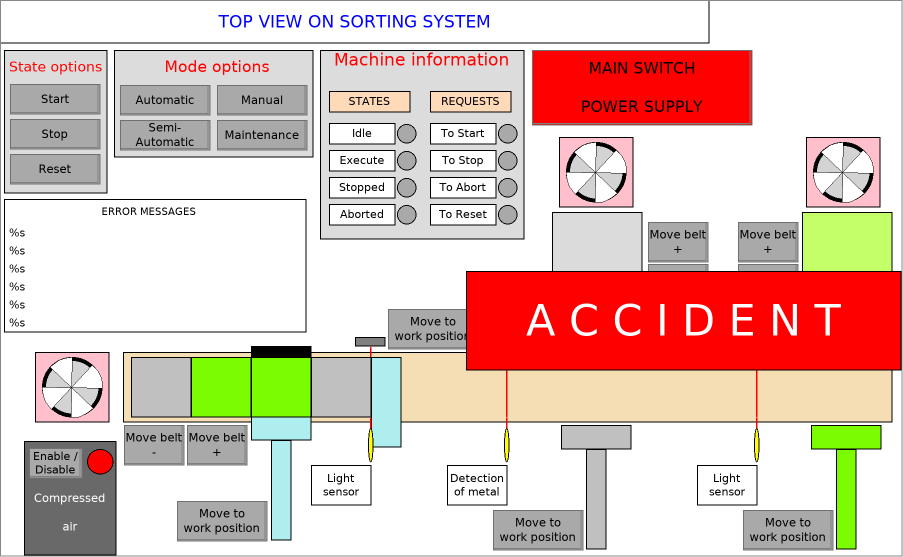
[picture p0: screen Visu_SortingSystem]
VISUALIZATION Visu_SortingSystem  // 903x557
    Rectangle (123,352 769x70)
    Rectangle (802,212 90x140)
    Rectangle (552,212 90x140)
    Rectangle (741,337 30x9)
    Rectangle (492,337 30x9)
    Ellipse (504,428 5x34)
    Ellipse (754,428 5x34)
    Group (562,426 70x124)
        p2738717112: MAIN.fbVisu.lrYMetal
        Rectangle (-1,-1 70x24)
        Rectangle (24,23 20x100)
    Group (812,426 70x124)
        p2738717112: MAIN.fbVisu.lrYPlastic
        Rectangle (-1,-1 70x24)
        Rectangle (24,23 20x100)
    Group (252,417 60x124)
        p2738717112: MAIN.fbVisu.lrYClamp
        Rectangle (19,23 20x100)
        Rectangle (-1,-1 60x24)
    Rectangle (131,357 60x60)
        p3560616238: MAIN.fbVisu.aBoxX[4]
        p2738717112: MAIN.fbVisu.aBoxY[4]
    Rectangle (251,357 60x60)
        p3560616238: MAIN.fbVisu.aBoxX[2]
        p2738717112: MAIN.fbVisu.aBoxY[2]
    Rectangle (191,357 60x60)
        p3560616238: MAIN.fbVisu.aBoxX[3]
        p2738717112: MAIN.fbVisu.aBoxY[3]
    Textfield (447,465 60x40), "Detection of metal"
    Textfield (697,465 60x40), "Light sensor"
    Rectangle (506,418 1x10)
    Rectangle (506,347 1x70), invisible if: MAIN.fbMetalSorting.fbSensorDelay.bInput
    Rectangle (756,347 1x70), invisible if: MAIN.fbVisu.bPlasticSensor
    Rectangle (756,418 1x10)
    Textfield (0,0 709x43), "TOP VIEW ON SORTING SYSTEM"
    Rectangle (4,50 103x143)
    Button (10,84 90x30), "Start", colour toggle: MAIN.fbVisu.bButtonColorStart, input disabled if: NOT MAIN.fbVisu.bButtonColorStart AND NOT MAIN.fbVisu.bAccident
        p573394764: MAIN.fbVisu.nButtonColorStart
        toggle MAIN.fbVisu.bButtonStartOut
    Button (10,119 90x30), "Stop", colour toggle: MAIN.fbVisu.bButtonColorStop, input disabled if: NOT MAIN.fbVisu.bButtonColorStop
        p573394764: MAIN.fbVisu.nButtonColorStop
        toggle MAIN.fbVisu.bButtonStopOut
    Button (10,154 90x30), "Reset", colour toggle: MAIN.fbVisu.bButtonColorReset, input disabled if: NOT MAIN.fbVisu.bButtonColorReset
        p573394764: MAIN.fbVisu.nButtonColorReset
        toggle MAIN.fbVisu.bButtonResetOut
    Textfield (7,54 98x25), "State options"
    Rectangle (114,50 199x107)
    Button (120,85 90x30), "Automatic", colour toggle: MAIN.fbVisu.bButtonColorAuto, input disabled if: NOT MAIN.fbVisu.bButtonColorAuto
        p573394764: MAIN.fbVisu.nButtonColorAuto
        toggle MAIN.fbVisu.bButtonAutoOut
    Button (217,85 90x30), "Manual", colour toggle: MAIN.fbVisu.bButtonColorManu, input disabled if: NOT MAIN.fbVisu.bButtonColorManu
        p573394764: MAIN.fbVisu.nButtonColorManu
        toggle MAIN.fbVisu.bButtonManuOut
    Button (120,120 90x30), "Semi- Automatic", colour toggle: MAIN.fbVisu.bButtonColorSemi, input disabled if: NOT MAIN.fbVisu.bButtonColorSemi
        p573394764: MAIN.fbVisu.nButtonColorSemi
        toggle MAIN.fbVisu.bButtonSemiOut
    Button (217,120 90x30), "Maintenance", colour toggle: MAIN.fbVisu.bButtonColorMaint, input disabled if: NOT MAIN.fbVisu.bButtonColorMaint
        p573394764: MAIN.fbVisu.nButtonColorMaint
        toggle MAIN.fbVisu.bButtonMaintenanceOut
    Textfield (156,52 122x29), "Mode options"
    Rectangle (24,441 92x114), "Compressed air"
    Ellipse (87,449 26x25), colour toggle: MAIN.fbVisu.bComprAirEnabled
    Button (648,222 60x40), "Move belt +", colour toggle: MAIN.fbVisu.bButtonColorMetalFw, invisible if: NOT (MAIN.fbVisu.bManual OR MAIN.fbVisu.bMaintenance), input disabled if: NOT MAIN.fbVisu.bButtonColorMetalFw
        p573394764: MAIN.fbVisu.nButtonColorMetalFw
        toggle MAIN.fbVisu.bButtonMetalFwOut
    Button (738,222 60x40), "Move belt +", colour toggle: MAIN.fbVisu.bButtonColorPlasticFw, invisible if: NOT (MAIN.fbVisu.bManual OR MAIN.fbVisu.bMaintenance), input disabled if: NOT MAIN.fbVisu.bButtonColorPlasticFw
        p573394764: MAIN.fbVisu.nButtonColorPlasticFw
        toggle MAIN.fbVisu.bButtonPlasticFwOut
    Button (187,425 60x40), "Move belt +", colour toggle: MAIN.fbVisu.bButtonColorMainFw, invisible if: NOT (MAIN.fbVisu.bManual OR MAIN.fbVisu.bMaintenance), input disabled if: NOT MAIN.fbVisu.bButtonColorMainFw
        p573394764: MAIN.fbVisu.nButtonColorMainFw
        toggle MAIN.fbVisu.bButtonMainFwOut
    Button (648,264 60x40), "Move belt -", colour toggle: MAIN.fbVisu.bButtonColorMetalBw, invisible if: NOT (MAIN.fbVisu.bManual OR MAIN.fbVisu.bMaintenance), input disabled if: NOT MAIN.fbVisu.bButtonColorMetalBw
        p573394764: MAIN.fbVisu.nButtonColorMetalBw
        toggle MAIN.fbVisu.bButtonMetalBwOut
    Button (738,264 60x40), "Move belt -", colour toggle: MAIN.fbVisu.bButtonColorPlasticBw, invisible if: NOT (MAIN.fbVisu.bManual OR MAIN.fbVisu.bMaintenance), input disabled if: NOT MAIN.fbVisu.bButtonColorPlasticBw
        p573394764: MAIN.fbVisu.nButtonColorPlasticBw
        toggle MAIN.fbVisu.bButtonPlasticBwOut
    Button (124,425 60x40), "Move belt -", colour toggle: MAIN.fbVisu.bButtonColorMainBw, invisible if: NOT (MAIN.fbVisu.bManual OR MAIN.fbVisu.bMaintenance), input disabled if: NOT MAIN.fbVisu.bButtonColorMainBw
        p573394764: MAIN.fbVisu.nButtonColorMainBw
        toggle MAIN.fbVisu.bButtonMainBwOut
    Button (388,309 90x40), "Move to work position", colour toggle: MAIN.fbVisu.bButtonColorBarrier, invisible if: NOT (MAIN.fbVisu.bManual OR MAIN.fbVisu.bMaintenance), input disabled if: NOT MAIN.fbVisu.bButtonColorBarrier
        p573394764: MAIN.fbVisu.nButtonColorBarrier
        toggle MAIN.fbVisu.bButtonBarrierToWorkOut
    Button (177,501 90x40), "Move to work position", colour toggle: MAIN.fbVisu.bButtonColorClamp, invisible if: NOT (MAIN.fbVisu.bManual OR MAIN.fbVisu.bMaintenance), input disabled if: NOT MAIN.fbVisu.bButtonColorClamp
        p573394764: MAIN.fbVisu.nButtonColorClamp
        toggle MAIN.fbVisu.bButtonClampToWorkOut
    Button (493,510 90x40), "Move to work position", colour toggle: MAIN.fbVisu.bButtonColorMetalCyl, invisible if: NOT (MAIN.fbVisu.bManual OR MAIN.fbVisu.bMaintenance), input disabled if: NOT MAIN.fbVisu.bButtonColorMetalCyl
        p573394764: MAIN.fbVisu.nButtonColorMetalCyl
        toggle MAIN.fbVisu.bButtonMetalToWorkOut
    Button (743,510 90x40), "Move to work position", colour toggle: MAIN.fbVisu.bButtonColorPlasticCyl, invisible if: NOT (MAIN.fbVisu.bManual OR MAIN.fbVisu.bMaintenance), input disabled if: NOT MAIN.fbVisu.bButtonColorPlasticCyl
        p573394764: MAIN.fbVisu.nButtonColorPlasticCyl
        toggle MAIN.fbVisu.bButtonPlasticToWorkOut
    Rectangle (371,357 30x90)
        p2738717112: MAIN.fbVisu.lrYBarrier
    Rectangle (355,337 30x9)
    Ellipse (368,428 5x34)
    Rectangle (370,418 1x10)
    Rectangle (370,347 1x70), invisible if: MAIN.fbVisu.bBarrierSensor
    Textfield (311,465 60x40), "Light sensor"
    Button (532,50 220x75), "MAIN SWITCH POWER SUPPLY", colour toggle: MAIN.fbVisu.bPowerEnabled
        toggle MAIN.fbVisu.bButtonPowerOut
    Rectangle (320,50 204x189), "Machine information"
    Textfield (329,123 66x21), "Idle"
    Textfield (329,150 66x21), "Execute"
    Textfield (329,177 66x21), "Stopped"
    Textfield (329,204 66x21), "Aborted"
    Textfield (430,123 66x21), "To Start"
    Textfield (430,150 66x21), "To Stop"
    Textfield (430,177 66x21), "To Abort"
    Textfield (430,204 66x21), "To Reset"
    Textfield (329,91 81x21), "STATES"
    Textfield (430,91 81x21), "REQUESTS"
    Ellipse (397,124 19x19), colour toggle: MAIN.fbVisu.bIdle
    Ellipse (397,151 19x19), colour toggle: MAIN.fbVisu.bStarted AND MAIN.fbVisu.bPowerEnabled
    Ellipse (397,178 19x19), colour toggle: MAIN.fbVisu.bStopped
    Ellipse (397,205 19x19), colour toggle: MAIN.fbVisu.bAborted
    Ellipse (498,124 19x19), colour toggle: MAIN.fbVisu.bButtonStartIn
    Ellipse (498,151 19x19), colour toggle: MAIN.fbVisu.bButtonStopIn
    Ellipse (498,205 19x19), colour toggle: MAIN.fbVisu.bReset
    Ellipse (498,178 19x19), colour toggle: MAIN.fbVisu.bButtonAbortIn
    Rectangle (251,346 60x11)
    Rectangle (311,357 60x60)
        p3560616238: MAIN.fbVisu.aBoxX[1]
        p2738717112: MAIN.fbVisu.aBoxY[1]
    Button (29,448 53x30), "Enable / Disable", colour toggle: MAIN.fbVisu.bButtonColorComprAir, invisible if: NOT MAIN.fbVisu.bMaintenance, input disabled if: NOT MAIN.fbVisu.bButtonColorComprAir
        p573394764: MAIN.fbVisu.nButtonColorComprAir
        toggle MAIN.fbVisu.bButtonComprAirOut
    Group (4,199 302x133)
        Rectangle (0,0 302x133)
        Textfield (72,3 146x19), "ERROR MESSAGES"
        Textfield (2,26 298x16), "%s", text variable: MAIN.fbVisu.sMessageMainAxis
        Textfield (2,44 298x16), "%s", text variable: MAIN.fbVisu.sMessageMetalAxis
        Textfield (2,62 298x16), "%s", text variable: MAIN.fbVisu.sMessagePlasticAxis
        Textfield (2,80 298x16), "%s", text variable: MAIN.fbVisu.sMessageClamp
        Textfield (2,98 298x16), "%s", text variable: MAIN.fbVisu.sMessageMetalCyl
        Textfield (2,116 298x16), "%s", text variable: MAIN.fbVisu.sMessagePlasticCyl
    Rectangle (466,271 435x99), "A C C I D E N T", invisible if: NOT MAIN.fbVisu.bAccident
    Textfield (35,352 74x70), invisible if: NOT MAIN.fbVisu.bMainAxisMoves
    Rectangle (71,357 1x60)
    Rectangle (42,387 60x1)
    Ellipse (42,357 60x60)
    Polygon (72,357) (71,417) (78,417) (83,415) (88,412) (93,408) (50,367) (47,371) (45,375) (43,380) (42,387) (102,388) (102,382) (101,377) (98,371) (92,365) (51,409) (48,405) (45,401) (43,395) (42,388) (43,382) (44,377) (47,371) (51,366) (55,363) (59,360) (65,358)
        p2858320360: MAIN.fbVisu.nAngleMain
    Textfield (559,137 74x70), invisible if: NOT MAIN.fbVisu.bMetalAxisMoves
    Rectangle (595,142 1x60)
    Rectangle (566,172 60x1)
    Ellipse (566,142 60x60)
    Polygon (596,142) (595,202) (602,202) (607,200) (612,197) (617,193) (574,152) (571,156) (569,160) (567,165) (566,172) (626,173) (626,167) (625,162) (622,156) (616,150) (575,194) (572,190) (569,186) (567,180) (566,173) (567,167) (568,162) (571,156) (575,151) (579,148) (583,145) (589,143)
        p2858320360: MAIN.fbVisu.nAngleMetal
    Textfield (806,137 74x70), invisible if: NOT MAIN.fbVisu.bPlasticAxisMoves
    Rectangle (842,142 1x60)
    Rectangle (813,172 60x1)
    Ellipse (813,142 60x60)
    Polygon (843,142) (842,202) (849,202) (854,200) (859,197) (864,193) (821,152) (818,156) (816,160) (814,165) (813,172) (873,173) (873,167) (872,162) (869,156) (863,150) (822,194) (819,190) (816,186) (814,180) (813,173) (814,167) (815,162) (818,156) (822,151) (826,148) (830,145) (836,143)
        p2858320360: MAIN.fbVisu.nAnglePlastic
END_VISUALIZATION
